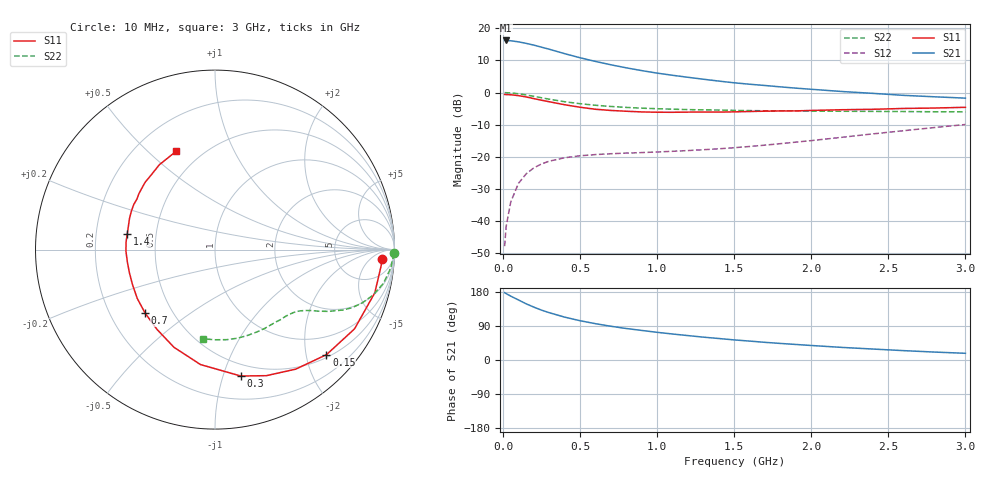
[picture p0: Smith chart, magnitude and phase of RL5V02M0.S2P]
!  SIEMENS Small Signal Semiconductors
! BFR93A , Si-NPN RF-Transistor in SOT23
!  Vce=5 V,  Ic=2 mA
! Common Emitter S-Parameters:  09. October 1995
#  GHz  S  MA  R  50
! f  S11  S21  S12  S22
! GHz  Mag  Ang  Mag  Ang  Mag  Ang  Mag  Ang
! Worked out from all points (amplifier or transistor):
!   30 points, 10 MHz to 3 GHz, reference 50 ohm
!   highest |S21| = 16.2 dB at 20 MHz (marker M1)
!   |S21| within 3 dB of that: start of sweep to 319.4 MHz
!   unconditionally stable (mu >= 1): 991.5 MHz to 2.608 GHz
!   at 200 MHz: K = 0.23, MSG = 19.1 dB, |S12| = -23.4 dB
!   at 1.1 GHz: K = 1.06, MAG = 10.3 dB, |S12| = -18.3 dB
!   at 3 GHz: K = 0.92, MSG = 4.1 dB, |S12| = -9.9 dB
!   S11 on the Smith chart (normalised r, x): 10 MHz: 18, -14; 150 MHz: 0.56, -2.41; 300 MHz: 0.39, -1.15; 700 MHz: 0.35, -0.35; 1.4 GHz: 0.34, +0.08; 3 GHz: 0.37, +0.62
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0.01  0.9334 -3.1  6.434 177.7  0.0041 88.7  0.996 -1.2
0.02  0.9291 -6.0  6.439 175.3  0.0083 85.0  0.9937 -2.3
0.05  0.9224 -15.1  6.365 168.5  0.02 81.4  0.9849 -5.9
0.1  0.8941 -29.6  6.127 158.4  0.0388 73.4  0.9573 -11.3
0.15  0.8535 -43.3  5.801 148.2  0.0546 65.9  0.9163 -16.1
0.2  0.8036 -56.0  5.445 139.5  0.0676 60.1  0.8724 -19.9
0.25  0.7586 -67.8  5.061 131.5  0.0778 54.5  0.829 -23.0
0.3  0.7188 -78.5  4.701 124.8  0.0858 50.7  0.7877 -25.3
0.4  0.6455 -97.2  4.012 113.1  0.097 44.6  0.7193 -28.6
0.5  0.5903 -112.8  3.465 103.6  0.1041 40.9  0.6697 -30.8
0.6  0.5492 -126.2  3.04 95.8  0.1086 38.7  0.6338 -32.4
0.7  0.5264 -137.6  2.695 89.0  0.1119 37.9  0.607 -34.0
0.8  0.5116 -147.8  2.417 83.1  0.1145 37.9  0.5871 -35.5
0.9  0.4994 -157.0  2.189 78.0  0.1166 38.5  0.571 -37.1
1.1  0.4931 -171.9  1.852 68.6  0.1221 40.9  0.5509 -40.8
1.3  0.4974 175.0  1.609 60.3  0.1292 44.5  0.5377 -45.0
1.4  0.4965 169.7  1.505 56.7  0.1335 46.6  0.5339 -47.1
1.6  0.5072 159.9  1.345 49.9  0.1451 50.3  0.5237 -52.3
1.9  0.5182 147.1  1.169 41.0  0.1695 55.5  0.5166 -60.5
2.2  0.5404 136.2  1.036 33.2  0.2016 58.2  0.5114 -69.3
2.6  0.5655 123.2  0.903 24.7  0.2553 58.5  0.5061 -82.5
3  0.589 111.5  0.818 17.7  0.3185 55.7  0.5016 -97.5
